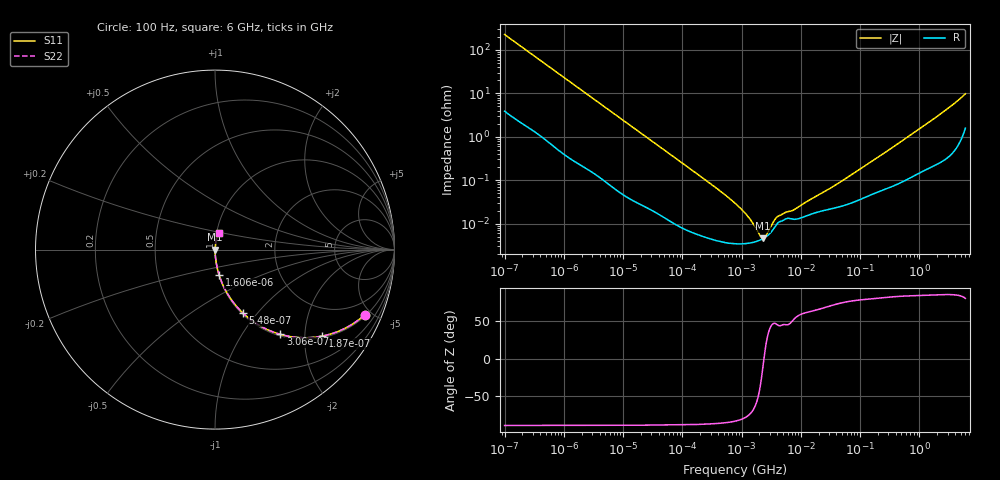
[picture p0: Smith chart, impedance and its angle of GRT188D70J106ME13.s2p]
!Murata Part Number: GRT188D70J106ME13
!These Parameters are Measured in Series Mode Connection
!Data Generated on Jun 19, 2026
!  o--ll--o
!Port1  Port2
!  o------o
!Operation Temp=25[degC], DC Bias Voltage=0[V]
!Freq. Start=100[Hz] Stop=6[GHz] 401[Steps]
# Hz S RI R 50
!Freq.(Hz) S11(Real) S11(Imag) S21(Real) S21(Imag) S12(Real) S12(Imag) S22(Real) S22(Imag)
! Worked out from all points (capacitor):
!   401 points, 100 Hz to 6 GHz, reference 50 ohm
!   read as one part in series: C = 6.96 uF near 109 Hz
!   lowest |Z| = 4.58 mohm at 2.269 MHz (marker M1)
!   series resonance near 2.387 MHz, so ESL is about 640 pH
!   S11 on the Smith chart (normalised r, x): 100 Hz: 1.08, -4.56; 187 Hz: 1.04, -2.45; 306 Hz: 1.03, -1.51; 548 Hz: 1.02, -0.85; 1.606 kHz: 1.01, -0.29; 6 GHz: 1.03, +0.19
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100  0.8344 -0.3633  0.1656 0.3633  0.1656 0.3633  0.8344 -0.3633
131  0.7496 -0.4249  0.2504 0.4249  0.2504 0.4249  0.7496 -0.4249
187  0.5985 -0.4816  0.4015 0.4816  0.4015 0.4816  0.5985 -0.4816
306  0.3642 -0.4722  0.6358 0.4722  0.6358 0.4722  0.3642 -0.4722
548  0.1567 -0.3548  0.8433 0.3548  0.8433 0.3548  0.1567 -0.3548
897  0.0671 -0.2418  0.9329 0.2418  0.9329 0.2418  0.0671 -0.2418
1606  0.0233 -0.1424  0.9767 0.1424  0.9767 0.1424  0.0233 -0.1424
2008  0.0156 -0.1151  0.9844 0.1151  0.9844 0.1151  0.0156 -0.1151
6433  0.00208 -0.037  0.9979 0.037  0.9979 0.037  0.00208 -0.037
40335  0.000199 -0.00605  0.9998 0.00605  0.9998 0.00605  0.000199 -0.00605
330837  4.3e-05 -0.000746  1 0.000746  1 0.000746  4.3e-05 -0.000746
774597  3.43e-05 -0.000293  1 0.000293  1 0.000293  3.43e-05 -0.000293
1585629  3.7e-05 -9e-05  1 9e-05  1 9e-05  3.7e-05 -9e-05
2268635  4.45e-05 -1.09e-05  1 1.09e-05  1 1.09e-05  4.45e-05 -1.09e-05
3245845  6.67e-05 6.75e-05  0.9999 -6.75e-05  0.9999 -6.75e-05  6.67e-05 6.75e-05
4246196  0.000108 0.000105  0.9999 -0.000105  0.9999 -0.000105  0.000108 0.000105
7599586  0.000125 0.000164  0.9999 -0.000164  0.9999 -0.000164  0.000125 0.000164
1.555665e7  0.000168 0.000339  0.9998 -0.000339  0.9998 -0.000339  0.000168 0.000339
4.165952e7  0.000237 0.000791  0.9998 -0.000791  0.9998 -0.000791  0.000237 0.000791
3.124326e8  0.000699 0.00501  0.9993 -0.00501  0.9993 -0.00501  0.000699 0.00501
2.048624e9  0.00326 0.0299  0.9967 -0.0299  0.9967 -0.0299  0.00326 0.0299
6e9  0.0244 0.0928  0.9756 -0.0928  0.9756 -0.0928  0.0244 0.0928
